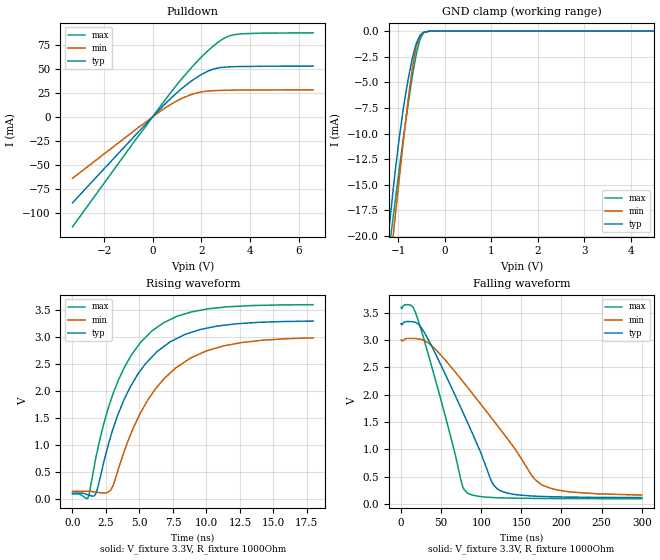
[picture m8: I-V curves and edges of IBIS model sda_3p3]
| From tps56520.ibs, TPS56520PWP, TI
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|   sda_3p3 Model
[Model]   sda_3p3
Model_type   I/O_open_drain
Polarity   Non-Inverting
Vinl = 0.6
Vinh = 1.8
Vmeas = 1.65
Vref = 3.3
Cref = 2pF
Rref = 1000
|   typ   min   max
|   (nom PVT)   (fast PVT)   (slow PVT)
C_comp   3.062e-13   2.486e-13   3.962e-13
| Where nom  PVT is Nominal Process, 3.3V, 27C
|   Fast PVT is Strong Process,  3.6V, -40C
|   Slow PVT is Weak Process,   3V, 125C
[Voltage Range]   3.3   3   3.6
|Junction Temperature
[Temperature Range]   27   125   -40
[Pullup Reference]   3.3   3   3.6
[Pulldown Reference]   0   0   0
[Power Clamp Reference]   3.3   3   3.6
[GND Clamp Reference]   0   0   0
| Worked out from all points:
|   slope of the pulldown table from 0 to 0.495 V, typ, clamps not added: 38 ohm
|   GND clamp passes 1 mA (typ) near -0.59 V on its own axis
|   falling waveform, V_fixture 3.3V, R_fixture 1000Ohm: 20-80 % time 58.4ns typ, 87.5ns min, 38.4ns max; typ from 3.3 V to 0.12 V
|   rising waveform, V_fixture 3.3V, R_fixture 1000Ohm: 20-80 % time 3.63ns typ, 4.02ns min, 3.3ns max; typ from 0.117 V to 3.29 V
[Pulldown]
|   Voltage   I(typ)   I(min)   I(max)
-3.3V     -89.61mA   -64.07mA   -114.6mA
-522mV    -13.85mA   -9.795mA   -17.48mA
705mV     18.33mA    12.41mA    24.11mA
1.161V    28.74mA    18.75mA    38.56mA
1.647V    38.31mA    23.73mA    52.8mA
2.103V    45.49mA    26.38mA    64.84mA
2.554V    50.15mA    27.32mA    75.07mA
2.832V    51.46mA    27.57mA    80.23mA
3.09V     51.99mA    27.71mA    83.75mA
3.623V    52.44mA    27.89mA    86.51mA
6.6V      52.88mA    28.18mA    87.54mA
[GND Clamp]
|   Voltage   I(typ)   I(min)   I(max)
-3.3V     -120.8mA   -120.7mA   -127.2mA
-1.206V   -19.53mA   -24.19mA   -21.62mA
-1.095V   -14.83mA   -19.32mA   -17.58mA
-990mV    -10.8mA    -14.82mA   -13.86mA
-894.3mV  -7.646mA   -10.86mA   -10.58mA
-788.7mV  -4.734mA   -6.748mA   -7.144mA
-686.4mV  -2.447mA   -3.316mA   -4.117mA
-603.6mV  -1.113mA   -1.363mA   -2.068mA
-524.4mV  -389.3uA   -458.8uA   -717.7uA
-448.8mV  -106.1uA   -150.6uA   -151.9uA
-267.3mV  -1.696uA   -6.404uA   -655.5nA
6.6V      0A         0A         0A
[POWER Clamp]
|   Voltage   I(typ)   I(min)   I(max)
-3.3V     0A         0A         0A
0V        0A         0A         0A
6.6V      0A         0A         0A
[Ramp]
R_load = 1000
|   typ   min   max
dV/dt_r   1.90982/3.65218e-09   1.71031/4.08492e-09   2.10018/3.30728e-09
dV/dt_f   1.9081/5.84321e-08   1.69999/8.74831e-08   2.0999/3.84167e-08
[Falling Waveform]
V_fixture = 3.3V
V_fixture_min = 3V
V_fixture_max = 3.6V
R_fixture = 1000Ohm
|   Time   V(typ)   V(min)   V(max)
0s        3.3V       3V         3.6V
11.56ns   3.338V     3.031V     3.643V
17.97ns   3.324V     3.028V     3.506V
37.22ns   2.916V     2.911V     2.57V
76.64ns   1.695V     2.251V     330.8mV
82.13ns   1.517V     2.15V      212mV
113.6ns   392.2mV    1.56V      121.8mV
125.1ns   237.1mV    1.34V      115.1mV
178ns     140mV      336.7mV    104mV
300ns     119.8mV    166.7mV    100.2mV
[Rising Waveform]
V_fixture = 3.3V
V_fixture_min = 3V
V_fixture_max = 3.6V
R_fixture = 1000Ohm
|   Time   V(typ)   V(min)   V(max)
0s        117mV      149.5mV    99.71mV
1.212ns   79.92mV    149.8mV    63.38mV
1.729ns   97.93mV    134.2mV    745.6mV
2.844ns   1.154V     168.8mV    1.815V
4.284ns   2.064V     1.165V     2.618V
5.915ns   2.627V     1.941V     3.11V
7.686ns   2.96V      2.425V     3.369V
10.01ns   3.162V     2.744V     3.516V
12.63ns   3.251V     2.898V     3.572V
17.97ns   3.294V     2.984V     3.598V
